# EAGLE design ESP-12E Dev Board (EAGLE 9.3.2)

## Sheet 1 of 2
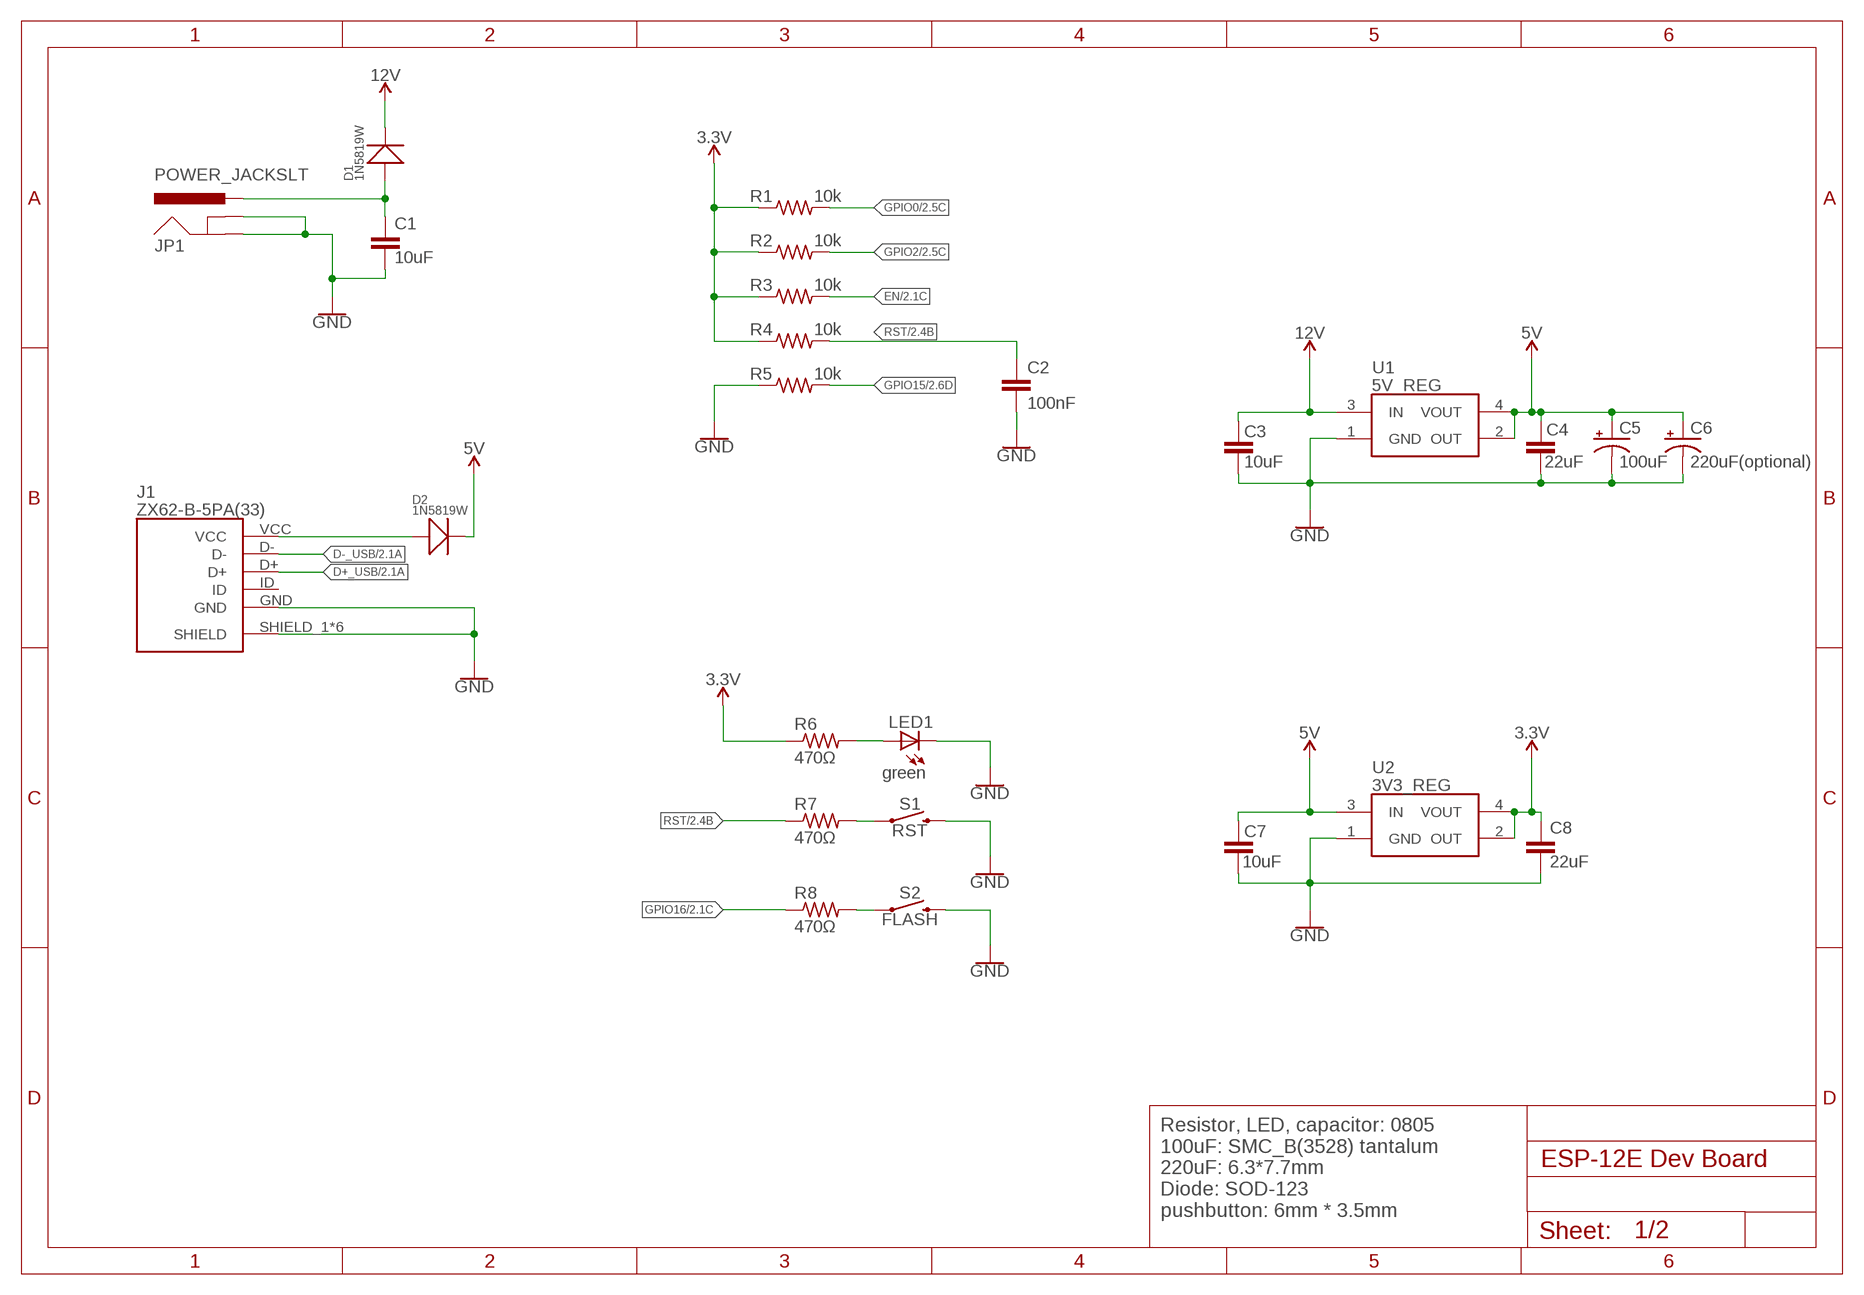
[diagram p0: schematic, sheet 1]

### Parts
C1  10uF  C-EUC0805  [C0805]
C2  100nF  C-EUC0805  [C0805]
C3  10uF  C-EUC0805  [C0805]
C4  22uF  C-EUC0805  [C0805]
C5  100uF  CPOL-USSMCB  [SMC_B]
C6  220uF(optional)  CPOL-USUD-6,3X7,7  [UD-6,3X7,7_NICHICON]
C7  10uF  C-EUC0805  [C0805]
C8  22uF  C-EUC0805  [C0805]
D1  1N5819W  SMD-DIODE-SCHOTTKY-20V-500MA(SOD-123)  [SOD-123]
D2  1N5819W  SMD-DIODE-SCHOTTKY-20V-500MA(SOD-123)  [SOD-123]
J1  ZX62-B-5PA(33)  [ZX62B5PA33]
JP1  POWER_JACKSLT  [POWER_JACK_SLOT]
LED1  green  LEDCHIP-LED0805  [CHIP-LED0805]
R1  10k  R-US_R0805  [R0805]
R2  10k  R-US_R0805  [R0805]
R3  10k  R-US_R0805  [R0805]
R4  10k  R-US_R0805  [R0805]
R5  10k  R-US_R0805  [R0805]
R6  470Ω  R-US_R0805  [R0805]
R7  470Ω  R-US_R0805  [R0805]
R8  470Ω  R-US_R0805  [R0805]
S1  RST  MOMENTARY-SWITCH-SPST-SMD-6.0X3.5MM  [TACTILE_SWITCH_SMD_6.0X3.5MM]
S2  FLASH  MOMENTARY-SWITCH-SPST-SMD-6.0X3.5MM  [TACTILE_SWITCH_SMD_6.0X3.5MM]
U1  5V_REG  AZ1117H-5.0TRE1  [SOT230P700X170-4N]
U2  3V3_REG  AZ1117H-5.0TRE1  [SOT230P700X170-4N]

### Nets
3.3V [power]: C8.2 R1.1 R2.1 R3.1 R4.1 R6.1 U2.2(OUT) U2.4(VOUT) ; also sheet 2
5V [power]: C4.1 C5.+ C6.+ C7.1 D2.- U1.2(OUT) U1.4(VOUT) U2.3(IN) ; also sheet 2
5V_INPUT [power]: D2.+ J1.VCC
12V [power]: C3.1 D1.- U1.3(IN) ; also sheet 2
D+_USB: J1.D+ ; also sheet 2
D-_USB: J1.D- ; also sheet 2
EN: R3.2 ; also sheet 2
GND [power]: C1.1 C2.1 C3.2 C4.2 C5.- C6.- C7.2 C8.1 J1.GND J1.SHIELD_1(SHIELD) J1.SHIELD_2(SHIELD) J1.SHIELD_3(SHIELD) J1.SHIELD_4(SHIELD) J1.SHIELD_5(SHIELD) J1.SHIELD_6(SHIELD) JP1.GND@1(GNDBREAK) JP1.GND@2(GND) LED1.C R5.1 S1.2 S2.2 U1.1(GND) U2.1(GND) ; also sheet 2
GPIO0: R1.2 ; also sheet 2
GPIO2: R2.2 ; also sheet 2
GPIO15: R5.2 ; also sheet 2
GPIO16: R8.1 ; also sheet 2
N$3: C1.2 D1.+ JP1.PWR
N$4: LED1.A R6.2
POWER: R7.2 S1.1
POWER1: R8.2 S2.1
RST: C2.2 R4.2 R7.1 ; also sheet 2
Unconnected: J1.ID

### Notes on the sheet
- Resistor, LED, capacitor: 0805
  100uF: SMC_B(3528) tantalum
  220uF: 6.3*7.7mm
  Diode: SOD-123
  pushbutton: 6mm * 3.5mm

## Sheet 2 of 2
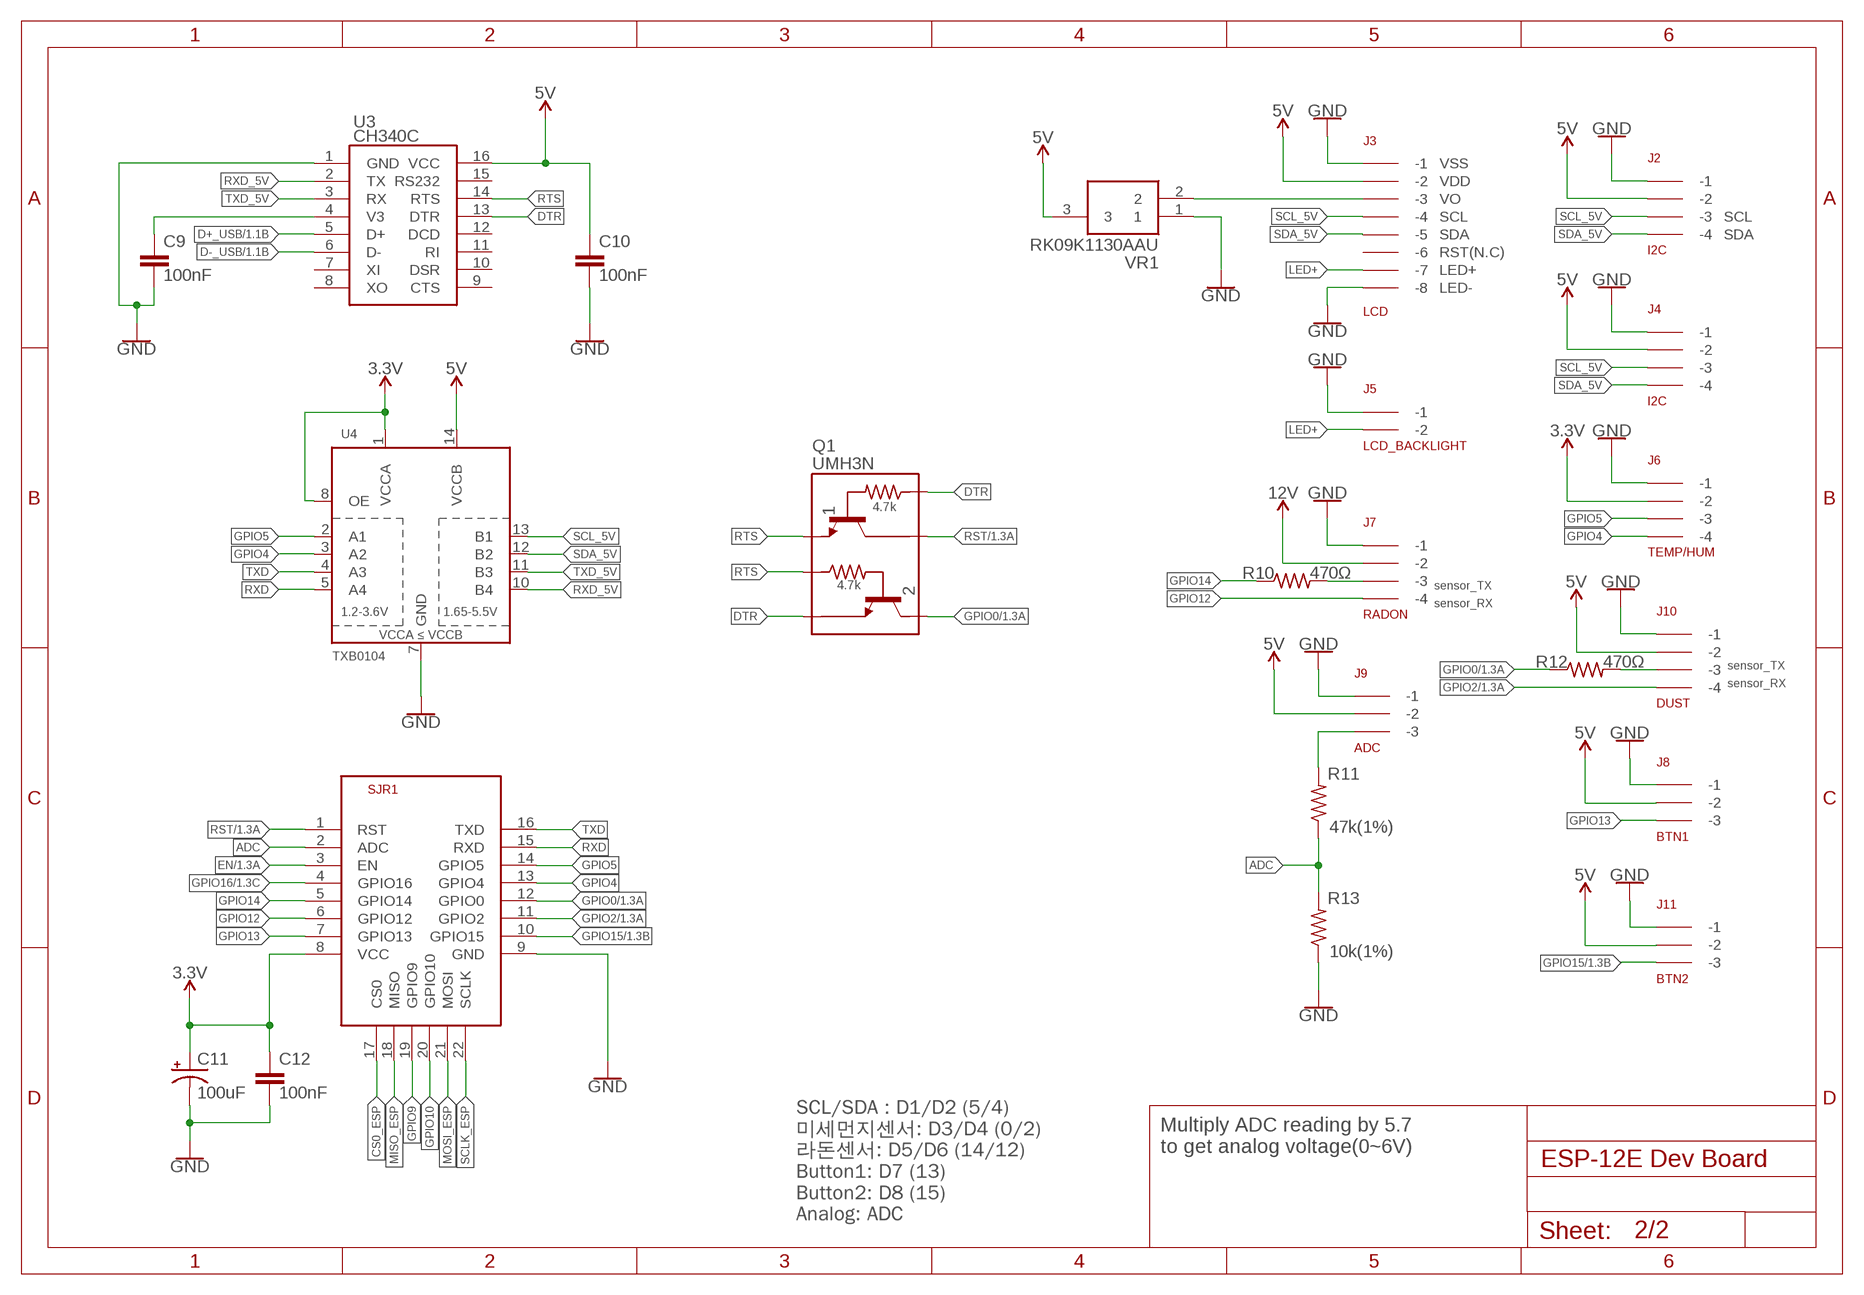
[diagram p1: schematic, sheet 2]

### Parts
C9  100nF  C-EUC0805  [C0805]
C10  100nF  C-EUC0805  [C0805]
C11  100uF  CPOL-USSMCB  [SMC_B]
C12  100nF  C-EUC0805  [C0805]
J2  I2C  5267-4  [5267-4]
J3  LCD  5267-8  [5267-8]
J4  I2C  5267-4  [5267-4]
J5  LCD_BACKLIGHT  5267-2  [5267-2]
J6  TEMP/HUM  5267-4  [5267-4]
J7  RADON  5267-4  [5267-4]
J8  BTN1  5267-3  [5267-3]
J9  ADC  5267-3  [5267-3]
J10  DUST  5267-4  [5267-4]
J11  BTN2  5267-3  [5267-3]
Q1  UMH3N  UMH3NFHATN  [SOT65P210X100-6N]
R10  470Ω  R-US_R0805  [R0805]
R11  47k(1%)  R-US_R0805  [R0805]
R12  470Ω  R-US_R0805  [R0805]
R13  10k(1%)  R-US_R0805  [R0805]
SJR1  ESP-12E  ESP8266-12EESP12E  [ESP8266-ESP12E]
U3  CH340C  CH340G  [SOIC16]
U4  TXB0104  TXB0104PWR  [TSSOP14]
VR1  RK09K1130AAU  RK09K1130A6S  [RK09K1130BGM]

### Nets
3.3V [power]: C11.+ C12.2 J6.P$2(-2) SJR1.8(VCC) U4.1(VCCA) U4.8(OE) ; also sheet 1
5V [power]: C10.2 J2.P$2(-2) J3.P$2(-2) J4.P$2(-2) J8.P$2(-2) J9.P$2(-2) J10.P$2(-2) J11.P$2(-2) U3.16(VCC) U4.14(VCCB) VR1.3 ; also sheet 1
12V [power]: J7.P$2(-2) ; also sheet 1
ADC: R11.1 R13.2 SJR1.2(ADC)
CS0_ESP: SJR1.17(CS0)
D+_USB: U3.5(D+) ; also sheet 1
D-_USB: U3.6(D-) ; also sheet 1
DTR: Q1.2 Q1.4 U3.13(DTR)
EN: SJR1.3(EN) ; also sheet 1
GND [power]: C9.1 C10.1 C11.- C12.1 J2.P$1(-1) J3.P$1(-1) J3.P$8(-8) J4.P$1(-1) J5.P$1(-1) J6.P$1(-1) J7.P$1(-1) J8.P$1(-1) J9.P$1(-1) J10.P$1(-1) J11.P$1(-1) R13.1 SJR1.9(GND) U3.1(GND) U4.7(GND) VR1.1 ; also sheet 1
GPIO0: Q1.3 R12.1 SJR1.12(GPIO0) ; also sheet 1
GPIO2: J10.P$4(-4) SJR1.11(GPIO2) ; also sheet 1
GPIO4: J6.P$4(-4) SJR1.13(GPIO4) U4.3(A2)
GPIO5: J6.P$3(-3) SJR1.14(GPIO5) U4.2(A1)
GPIO9: SJR1.19(GPIO9)
GPIO10: SJR1.20(GPIO10)
GPIO12: J7.P$4(-4) SJR1.6(GPIO12)
GPIO13: J8.P$3(-3) SJR1.7(GPIO13)
GPIO14: R10.1 SJR1.5(GPIO14)
GPIO15: J11.P$3(-3) SJR1.10(GPIO15) ; also sheet 1
GPIO16: SJR1.4(GPIO16) ; also sheet 1
LED+: J3.P$7(-7) J5.P$2(-2)
MISO_ESP: SJR1.18(MISO)
MOSI_ESP: SJR1.21(MOSI)
N$1: C9.2 U3.4(V3)
N$2: J3.P$3(-3) VR1.2
N$5: J9.P$3(-3) R11.2
N$6: J7.P$3(-3) R10.2
N$9: J10.P$3(-3) R12.2
RST: Q1.6 SJR1.1(RST) ; also sheet 1
RTS: Q1.1 Q1.5 U3.14(RTS)
RXD: SJR1.15(RXD) U4.5(A4)
RXD_5V: U3.2(TX) U4.10(B4)
SCL_5V: J2.P$3(-3) J3.P$4(-4) J4.P$3(-3) U4.13(B1)
SCLK_ESP: SJR1.22(SCLK)
SDA_5V: J2.P$4(-4) J3.P$5(-5) J4.P$4(-4) U4.12(B2)
TXD: SJR1.16(TXD) U4.4(A3)
TXD_5V: U3.3(RX) U4.11(B3)
Unconnected: J3.P$6(-6) U3.7(XI) U3.8(XO) U3.9(CTS) U3.10(DSR) U3.11(RI) U3.12(DCD) U3.15(RS232)

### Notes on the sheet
- VSS
- VDD
- VO
- SCL | SCL
- SDA | SDA
- RST(N.C)
- LED+
- LED-
- sensor_TX
- sensor_RX
- sensor_TX
- sensor_RX
- SCL/SDA : D1/D2 (5/4)
  미세먼지센서: D3/D4 (0/2)
  라돈센서: D5/D6 (14/12)
  Button1: D7 (13)
  Button2: D8 (15)
  Analog: ADC
- Multiply ADC reading by 5.7
  to get analog voltage(0~6V)

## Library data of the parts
C1-C4 C7-C10 C12 = rcl:C-EU: CAPACITOR, European symbol; SPICEPREFIX: C
C5 C6 C11 = rcl:CPOL-US: POLARIZED CAPACITOR, American symbol; SPICEPREFIX: C
D1 D2 = Seeed-Diode:SMD-DIODE-SCHOTTKY-20V-500MA(SOD-123): 304020032; MPN: SS0520-7-F; VALUE: 20V-500MA
J1 = SamacSys_Parts:ZX62-B-5PA(33): USB Connectors MICRO B RECEPT RA SMT BTTM MNT Source: Datasheet; DESCRIPTION: USB Connectors MICRO B RECEPT RA SMT BTTM MNT; HEIGHT: 2.8mm; MANUFACTURER_NAME: Hirose; MANUFACTURER_PART_NUMBER: ZX62-B-5PA(33); MOUSER_PART_NUMBER: 798-ZX62-B-5PA33; MOUSER_PRICE-STOCK: https://www.mouser.com/Search/Refine.aspx?Keyword=798-ZX62-B-5PA33
J2 J4 J6 J7 J10 = con-molex-spox:5267-4
J3 = con-molex-spox:5267-8
J5 = con-molex-spox:5267-2
J8 J9 J11 = con-molex-spox:5267-3
JP1 = kanflo:POWER_JACK: Power Jack This is the standard 5.5mm barrel jack for power. The SLT footprint has been proven in designs produced by DirtyPCBs.com and only works if the mill layer is transmitted to the PCB fab house and the fab house accepts it. Rumours has it OSH Park accepts this design too. This symbol is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
LED1 = adafruit:LED: LED
Q1 = SamacSys_Parts:UMH3NFHATN: ROHM - UMH3NFHATN - TRANS, NPN, AUTO, 4.7K/4.7K, SOT-353 Source: Datasheet; DESCRIPTION: ROHM - UMH3NFHATN - TRANS, NPN, AUTO, 4.7K/4.7K, SOT-353; HEIGHT: 1mm; MANUFACTURER_NAME: ROHM Semiconductor; MANUFACTURER_PART_NUMBER: UMH3NFHATN; MOUSER_PART_NUMBER: 755-UMH3NFHATN; MOUSER_PRICE-STOCK: https://www.mouser.com/Search/Refine.aspx?Keyword=755-UMH3NFHATN
R1-R8 R10-R13 = rcl:R-US_: RESISTOR, American symbol; SPICEPREFIX: R
S1 S2 = SparkFun-Switches:MOMENTARY-SWITCH-SPST: Momentary Switch (Pushbutton) - SPST; PROD_ID: SWCH-00815; SF_SKU: COM-08229
SJR1 = esp12e:ESP8266-12E: ESP8266-12E Library for Eagle CAD The author not responsible for any damages or errors!. Created by Suhail jr.lt;/author>
U1 U2 = SamacSys_Parts:AZ1117H-5.0TRE1: 1A 5V LDO Linear Voltage Reg SOT-223 Diodes Inc AZ1117H-5.0TRE1, Single Linear Voltage Regulator, 1A 4.9 5.1 V, 1%, 3-Pin SOT-223 Source: Datasheet; DESCRIPTION: 1A 5V LDO Linear Voltage Reg SOT-223 Diodes Inc AZ1117H-5.0TRE1, Single Linear Voltage Regulator, 1A 4.9 5.1 V, 1%, 3-Pin SOT-223; HEIGHT: 1.7mm; MANUFACTURER_NAME: Diodes Inc.; MANUFACTURER_PART_NUMBER: AZ1117H-5.0TRE1; MOUSER_PART_NUMBER: 621-AZ1117H-5.0TRE1; MOUSER_PRICE-STOCK: https://www.mouser.com/Search/Refine.aspx?Keyword=621-AZ1117H-5.0TRE1
U3 = ch340g:CH340G
U4 = SparkFun-IC-Comms:TXB0104PWR: 4-Bit Bi-Directional Level Shifter 1.2V-3.6V (VCCA) to 1.65V-5.5V (VCCB) bi-directional level shifter with auto direction sensing. Max data rate - VCCA 1.8V: 20Mbps (50ns), VCCA 3.3V: 100Mbps (10ns) Digikey: 296-21929-1-ND (TSSOP) Datasheet SparkFun Products SparkFun Cellular Shield - MG2639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; PROD_ID: NA-XXXXX
VR1 = SamacSys_Parts:RK09K1130A6S: Audio single pot. 10K Vertical 15mm,1B Alps RK09K Series, Linear Potentiometer with a 6 mm Dia. Shaft, 10k, +/-20%, Through Hole Source: Datasheet; DESCRIPTION: Audio single pot. 10K Vertical 15mm,1B Alps RK09K Series, Linear Potentiometer with a 6 mm Dia. Shaft, 10k, +/-20%, Through Hole; HEIGHT: mm; MANUFACTURER_NAME: ALPS; MANUFACTURER_PART_NUMBER: RK09K1130A6S; MOUSER_PART_NUMBER: 688-RK09K1130A6S; MOUSER_PRICE-STOCK: https://www.mouser.com/Search/Refine.aspx?Keyword=688-RK09K1130A6S

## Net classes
1 power: width 0.457 mm

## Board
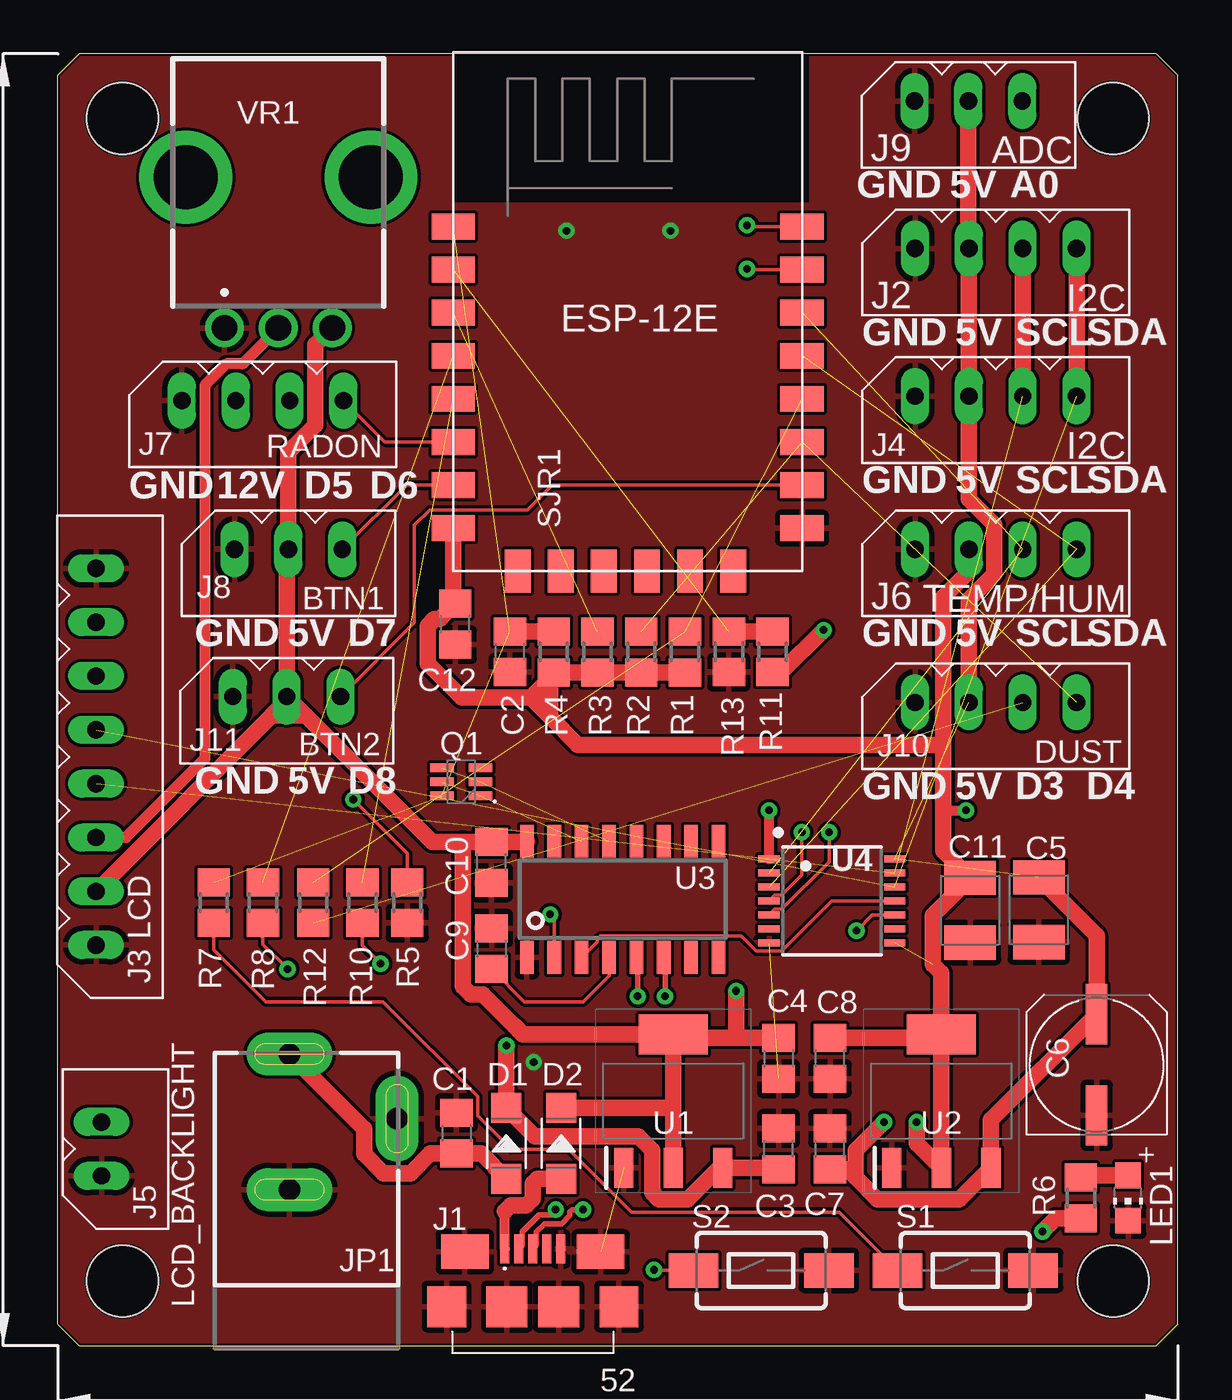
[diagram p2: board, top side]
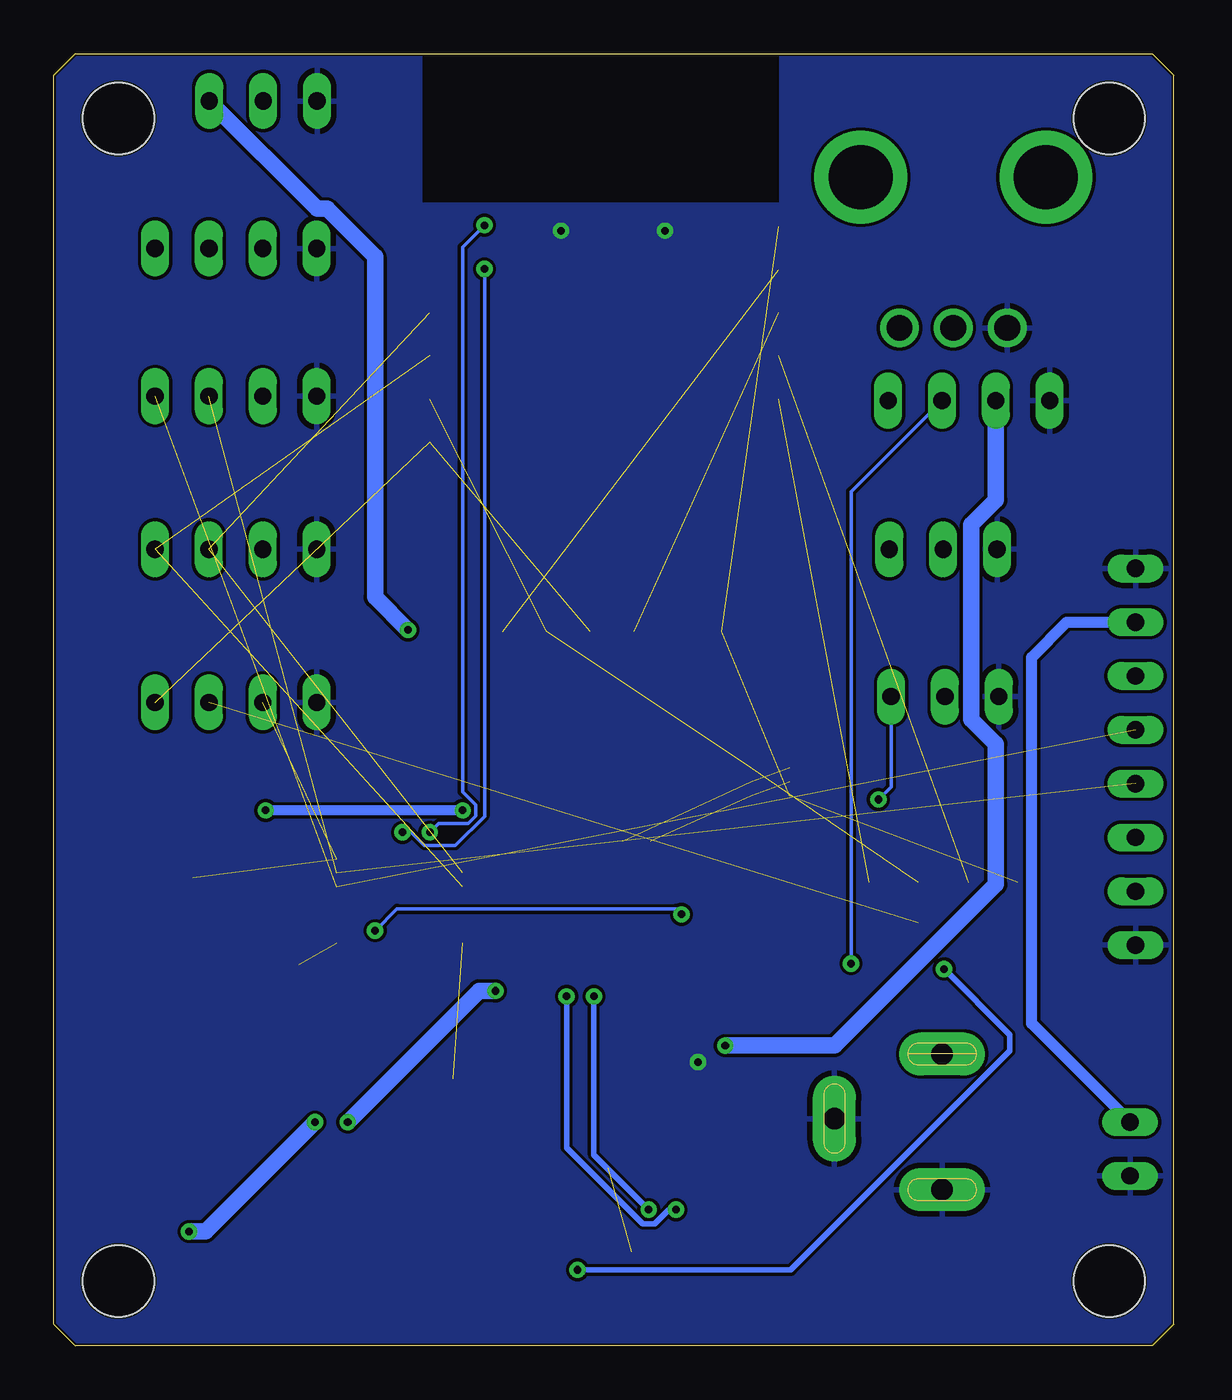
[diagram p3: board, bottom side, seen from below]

Size 52 x 60 mm. Coordinates in mm from the lower left corner, seen from the top.
Outline: 0,1 0,59 1,60 51,60 52,59 52,1 51,0 1,0 0,1
Copper layers (1*16): Top 0.035mm / dielectric 1.5mm / Bottom 0.035mm
Design rules "default *": minimum track width 6mil, minimum drill 0.35mm, track to track 6mil, track to pad 6mil, pad to pad 6mil, via to via 6mil, smd to smd 6mil, copper to edge 4mil, drill to drill 6mil, minimum pad ring 10mil, minimum via ring 8mil, stop-mask expansion 4mil, vias tented up to drill 0mil, thermal gap 10mil
Holes 3.3 mm at 3,57 49,57 49,3 3,3

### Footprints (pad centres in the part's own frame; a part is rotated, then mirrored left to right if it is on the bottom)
C0805 = smd 1.3 x 1.5: 1 -0.95,0; 2 0.95,0
SMC_B = smd 1.6 x 2.4: + -1.5,0; - 1.5,0
UD-6,3X7,7_NICHICON = smd 2.8 x 1: + 2.35,0; - -2.35,0
SOD-123 = smd 1.397 x 1.397: + -1.651,0; - 1.651,0
ZX62B5PA33 = smd 0.4 x 1.35: D+ 0,1.95; D- -0.65,1.95; GND 1.3,1.95; ID 0.65,1.95; VCC -1.3,1.95 | smd 2.2 x 1.6: SHIELD_1 -3.15,1.825; SHIELD_6 3.15,1.825 | smd 1.8 x 1.9: SHIELD_2 -4,-0.725; SHIELD_5 4,-0.725 | smd 1.9 x 1.9: SHIELD_3 -1.2,-0.725; SHIELD_4 1.2,-0.725
5267-4 = drill 0.8 long: P$1 0,0; P$2 2.5,0; P$3 5,0; P$4 7.5,0
5267-8 = drill 0.8 long: P$1 0,0; P$2 2.5,0; P$3 5,0; P$4 7.5,0; P$5 10,0; P$6 12.5,0; P$7 15,0; P$8 17.5,0
5267-2 = drill 0.8 long: P$1 0,0; P$2 2.5,0
5267-3 = drill 0.8 long: P$1 0,0; P$2 2.5,0; P$3 5,0
POWER_JACK_SLOT = drill 1 pad 2 long: GND@1 2.5,1.39; GND@2 -2.5,-1.91; PWR 2.5,-4.91
CHIP-LED0805 = smd 1.2 x 1.2: A 0,-1.05; C 0,1.05
SOT65P210X100-6N = smd 1.1 x 0.4: 1 -0.9,0.65; 2 -0.9,0; 3 -0.9,-0.65; 4 0.9,-0.65; 5 0.9,0; 6 0.9,0.65
R0805 = smd 1.3 x 1.5: 1 -0.95,0; 2 0.95,0
TACTILE_SWITCH_SMD_6.0X3.5MM = smd 2.3 x 1.6: 1 -3.15,0; 2 3.15,0
ESP8266-ESP12E = smd 2 x 1.2: 1 -7.62,5.84; 2 -7.62,3.84; 3 -7.62,1.84; 4 -7.62,-0.16; 5 -7.62,-2.16; 6 -7.62,-4.16; 7 -7.62,-6.16; 8 -7.62,-8.16; 9 8.58,-8.16; 10 8.58,-6.16; 11 8.58,-4.16; 12 8.58,-2.16; 13 8.58,-0.16; 14 8.58,1.84; 15 8.58,3.84; 16 8.58,5.84 | smd 1.2 x 2: 17 -4.62,-10.16; 18 -2.62,-10.16; 19 -0.62,-10.16; 20 1.38,-10.16; 21 3.38,-10.16; 22 5.38,-10.16
SOT230P700X170-4N = smd 1.85 x 0.9: 1 -3.1,2.3; 2 -3.1,0; 3 -3.1,-2.3 | smd 1.85 x 3.2: 4 3.1,0
SOIC16 = smd 0.635 x 1.524: 1 -4.445,-2.695; 2 -3.175,-2.695; 3 -1.905,-2.695; 4 -0.635,-2.695; 5 0.635,-2.695; 6 1.905,-2.695; 7 3.175,-2.695; 8 4.445,-2.695; 9 4.445,2.695; 10 3.175,2.695; 11 1.905,2.695; 12 0.635,2.695; 13 -0.635,2.695; 14 -1.905,2.695; 15 -3.175,2.695; 16 -4.445,2.695
TSSOP14 = smd 0.305 x 0.991: 1 -1.95,-2.918; 2 -1.3,-2.918; 3 -0.65,-2.918; 4 0,-2.918; 5 0.65,-2.918; 6 1.3,-2.918; 7 1.95,-2.918; 8 1.95,2.918; 9 1.3,2.918; 10 0.65,2.918; 11 0,2.918; 12 -0.65,2.918; 13 -1.3,2.918; 14 -1.95,2.918
RK09K1130BGM = drill 1.2 pad 1.8: 1 -2.5,-12.5; 2 0,-12.5; 3 2.5,-12.5 | drill 2.97 pad 4.3: 4 4.3,-5.5; 5 -4.3,-5.5

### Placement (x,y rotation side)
C1  18.51,9.87 270 top
C2  20.99,32.23 90 top
C3  33.46,9.14 90 top
C4  33.47,13.35 270 top
C5  45.55,20.25 270 top
C6  48.23,13.05 90 top
C7  35.85,9.14 90 top
C8  35.86,13.35 90 top
C9  20.14,18.44 270 top
C10  20.13,22.45 90 top
C11  42.36,20.22 270 top
C12  18.45,33.51 90 top
D1  20.83,9.4 90 top
D2  23.37,9.4 90 top
J1  22.05,2.54 0 top
J2  39.8,50.96 0 top
J3  1.78,18.6 90 top
J4  39.8,44.1 0 top
J5  2.03,7.89 90 top
J6  39.8,36.99 0 top
J7  5.76,43.9 0 top
J8  8.21,36.99 0 top
J9  39.78,57.81 0 top
J10  39.8,29.88 0 top
J11  8.13,30.15 0 top
JP1  13.26,8.64 180 top
LED1  49.69,6.86 180 top
Q1  18.73,26.19 180 top
R1  29.12,32.23 90 top
R2  27.09,32.23 90 top
R3  25.06,32.23 90 top
R4  23.02,32.23 90 top
R5  16.23,20.57 90 top
R6  47.5,6.86 90 top
R7  7.24,20.57 270 top
R8  9.53,20.57 270 top
R10  14.14,20.57 270 top
R11  33.19,32.23 270 top
R12  11.86,20.57 270 top
R13  31.16,32.23 90 top
S1  42.13,3.49 0 top
S2  32.65,3.49 0 top
SJR1  25.97,46.13 0 top
U1  28.57,11.37 90 top
U2  41.02,11.37 90 top
U3  26.23,20.73 0 top
U4  35.94,20.66 270 top
VR1  10.24,59.77 0 top

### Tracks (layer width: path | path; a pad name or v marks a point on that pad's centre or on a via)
3.3V  (via drill 0.35)  (1 unrouted)
  Top 0.457: 33.02,27.91 | U4.1 v33.02,24.86 | 41.11,24.86 v42.16,24.86
  Top 0.762: C8.2 40.85,14.3 U2.4 | U2.4 U2.2 39.88,9.41 v39.88,10.38 | SJR1.8 18.35,34.56 C12.2 17.73,33.74 17.48,33.74 17.17,33.43 17.17,31.69 18.76,30.09 21.96,30.09 | R4.1 23.15,31.28 | 23.15,31.28 R3.1 R2.1 R1.1 | U2.4 41.02,17.31 40.62,17.7 40.62,19.99 C11.+ 41.11,22.97 41.11,24.86 41.11,27.91 | J6.P$2 42.3,35.95 41.11,34.76 41.11,27.91 | 21.96,30.09 22.87,31 | 21.96,30.09 22.87,29.19 | 22.87,29.19 24.15,27.91 33.02,27.91 41.11,27.91 | 22.87,29.19 22.87,31 | 22.87,31 23.15,31.28 | v45.72,5.3 46.33,5.91 R6.1
  Bottom 0.457: v33.02,24.86 v42.16,24.86
  Bottom 0.762: v45.72,5.3 44.96,5.3 v39.88,10.38
5V  (via drill 0.35)  (2 unrouted)
  Top 0.762: J10.P$2 42.3,34.66 43.49,35.84 43.49,38.14 42.3,39.32 J4.P$2 J2.P$2 42.28,50.98 J9.P$2 | J11.P$2 10.63,36.91 J8.P$2 10.71,41.51 11.95,42.75 11.95,46.48 VR1.3 | C5.+ 48.23,19.07 C6.+ 43.32,10.49 U2.3 41.86,6.81 38.05,6.81 37.05,7.81 | C4.1 31.24,14.3 | 31.24,14.3 28.74,14.3 U1.4 | U1.4 28.57,11.14 | 28.57,11.14 U1.2 | C7.1 36.66,8.19 37.05,7.81 | D2.- 28.48,11.05 28.57,11.14 | J3.P$2 9.94,29.26 | 9.94,29.26 10.63,29.95 J11.P$2 | 18.8,23.4 17.38,23.4 11.51,29.26 | 18.8,23.4 C10.2 21.75,23.4 U3.16 | J11.P$2 11.51,29.26 | 11.51,29.26 9.94,29.26 | 18.85,23.34 18.8,23.4 | U1.4 21.59,14.47 21.21,14.85 21.18,14.85 19.73,16.31 19.17,16.31 18.8,16.68 18.8,23.4 | 37.05,7.81 37.05,9.08 v38.35,10.38 | v31.5,16.48 31.5,14.55 31.24,14.3
  Bottom 0.762: v31.5,16.48 32.26,16.48 v38.35,10.38
5V_INPUT
  Top 0.457: J1.VCC 20.75,6.24
  Top 0.762: D2.+ 22.26,7.75 22.06,7.55 22.06,6.83 21.75,6.51 21.02,6.51 20.75,6.24
12V  (via drill 0.35)
  Top 0.762: C3.1 33.39,8.27 U1.3 30.7,8.27 29.25,6.81 27.9,6.81 27.59,7.12 27.59,9.08 26.95,9.72 22.15,9.72 D1.- v20.83,13.94
  Bottom 0.762: v20.83,13.94 15.75,13.94 8.26,21.42 8.26,27.95 9.39,29.08 9.39,38.14 8.26,39.27 J7.P$2
ADC  (1 unrouted)
  Top 0.762: R11.1 R13.2
D+_USB  (via drill 0.35)
  Top 0.254: v26.92,16.22 26.92,17.98 U3.5 | v24.38,6.32 23.88,6.32 23.77,6.21 23.77,6.05 23.39,5.66 22.6,5.66 22.22,5.28 22.22,4.66 J1.D+
  Bottom 0.254: v24.38,6.32 26.92,8.86 v26.92,16.22
D-_USB  (via drill 0.35)
  Top 0.254: v28.19,16.22 28.19,17.98 U3.6 | v23.11,6.32 23.11,6.2 22.98,6.07 22.36,6.07 21.57,5.28 21.57,4.66 J1.D-
  Bottom 0.254: v23.11,6.32 23.45,6.32 24.11,5.66 24.66,5.66 28.19,9.2 v28.19,16.22
DTR  (2 unrouted)
EN  (1 unrouted)
GND  (via drill 0.35)  (2 unrouted)
  other vias: 22.1,13.18 23.62,51.78 28.45,51.78
  pour Top: -6.89,65.66 -6.89,-6.35 57.47,-6.35 57.47,65.66
  pour Bottom: -8.89,75.66 -8.89,-4.35 77.47,-4.35 77.47,75.66
GPIO0  (3 unrouted)
GPIO2  (2 unrouted)
GPIO4  (2 unrouted)
GPIO5  (2 unrouted)
GPIO12
  Top 0.152: J7.P$4 15.19,41.97 SJR1.6
GPIO13
  Top 0.152: J8.P$3 16.19,39.97 SJR1.7
GPIO14  (1 unrouted)
GPIO15  (via drill 0.35)
  Top 0.152: SJR1.10 22.96,39.97 21.79,38.8 17.26,38.8 16.56,38.1 16.56,33.58 J11.P$3 | v13.72,25.37 16.23,22.86 R5.2
  Bottom 0.152: v13.72,25.37 13.13,25.96 J11.P$3
GPIO16  (1 unrouted)
LED+
  Bottom 0.508: J5.P$2 6.6,14.96 6.6,31.97 4.97,33.6 J3.P$7
N$1
  Top 0.152: C9.2 21.66,15.97 24.38,15.97 25.59,17.18 U3.4
N$2
  Top 0.508: VR1.2 8.58,45.61 7.83,45.61 6.82,44.61 6.82,27.26 3.16,23.6 J3.P$3
N$3
  Top 0.762: JP1.PWR 14.22,10.08 14.22,8.91 15.12,8.01 16.39,8.01 17.3,8.92 C1.2 19.65,8.92 D1.+
N$4
  Top 0.762: R6.2 47.6,7.91 LED1.A
N$5  (via drill 0.35)
  Top 0.762: R11.2 33.6,31.28 v35.56,33.24
  Bottom 0.762: J9.P$3 39.77,52.8 39.31,52.8 37.08,50.58 37.08,34.77 v35.56,33.24
N$6  (via drill 0.35)
  Top 0.152: R10.2 14.14,18.59 v14.99,17.75
  Bottom 0.152: v14.99,17.75 14.99,39.67 J7.P$3
N$9  (1 unrouted)
POWER
  Top 0.152: 7.8,19.62 R7.2 7.24,18.38 9.65,15.97 15.09,15.97 19.49,11.57 19.49,10.67 21.04,9.12 23.73,9.12 26.64,6.2 36.28,6.2 S1.1
POWER1  (via drill 0.35)
  Top 0.152: R8.2 9.53,18.64 v10.67,17.49 | v27.69,3.52 27.72,3.49 S2.1
  Bottom 0.254: v27.69,3.52 17.78,3.52 7.62,13.68 7.62,14.45 v10.67,17.49
RST  (3 unrouted)
  Top 0.762: R4.2 C2.2
RTS  (2 unrouted)
RXD  (via drill 0.35)
  Top 0.152: U4.5 33.29,20.27 33.61,20.27 35.81,22.48 v35.81,23.84 | v32,50.01 32.04,49.97 SJR1.15
  Bottom 0.152: v35.81,23.84 35.4,23.84 34.8,23.24 33.35,23.24 32,24.59 v32,50.01
RXD_5V  (via drill 0.35)
  Top 0.152: v37.08,19.27 37.82,20 U4.10 | v22.86,20.03 23.05,19.84 U3.2
  Bottom 0.152: v22.86,20.03 23.11,20.29 36.07,20.29 v37.08,19.27
SCL_5V  (2 unrouted)
  Top 0.762: J2.P$3 J4.P$3
SDA_5V  (2 unrouted)
  Top 0.762: J4.P$4 J2.P$4
TXD  (via drill 0.35)
  Top 0.152: U4.4 33.29,20.92 33.61,20.92 34.54,21.86 v34.54,23.84 | v32,52.04 32.07,51.97 SJR1.16
  Bottom 0.152: v34.54,23.84 34.13,24.25 32.77,24.25 32.41,24.61 32.41,25.11 33.02,25.72 33.02,51.02 v32,52.04
TXD_5V
  Top 0.152: U3.3 25.05,18.76 25.05,18.9 25.18,19.03 31.73,19.03 32.43,18.32 33.61,18.32 35.94,20.66 U4.11

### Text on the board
tPlace: GND | 5V | A0 | GND | 5V | SCL | SDA | GND | 5V | SCL | SDA | GND | 12V | D5 | D6 | GND | 5V | D7 | GND | 5V | SCL | SDA | GND | 5V | D8 | GND | 5V | D3 | D4

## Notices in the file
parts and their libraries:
SparkFun-PowerSymbols: Licensing: Creative Commons ShareAlike 4.0 International - https://creativecommons.org/licenses/by-sa/4.0
